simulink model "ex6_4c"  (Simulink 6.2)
settings: Solver=ode45  SolverMode=SingleTasking  StartTime=0.0  StopTime=10.0  RelTol=1e-3  AbsTol=1e-6

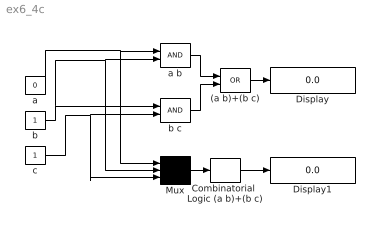
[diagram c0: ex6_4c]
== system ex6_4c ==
  (a b)+(b c) : Logic  Operator=OR
  Combinatorial  Logic (a b)+(b c) : CombinatorialLogic  TruthTable=[0;0;0;1;0;0;1;1]
  Display : Display
  Display1 : Display
  Mux : Mux  Inputs=3
  a : Constant  Value=0
  a b : Logic
  b : Constant
  b c : Logic
  c : Constant
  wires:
  a b/1 -> (a b)+(b c)/1
  b c/1 -> (a b)+(b c)/2
  (a b)+(b c)/1 -> Display/1
  b/1 -> b c/1, a b/2, Mux/2
  Mux/1 -> Combinatorial  Logic (a b)+(b c)/1
  Combinatorial  Logic (a b)+(b c)/1 -> Display1/1
  a/1 -> a b/1, Mux/1
  c/1 -> b c/2, Mux/3
